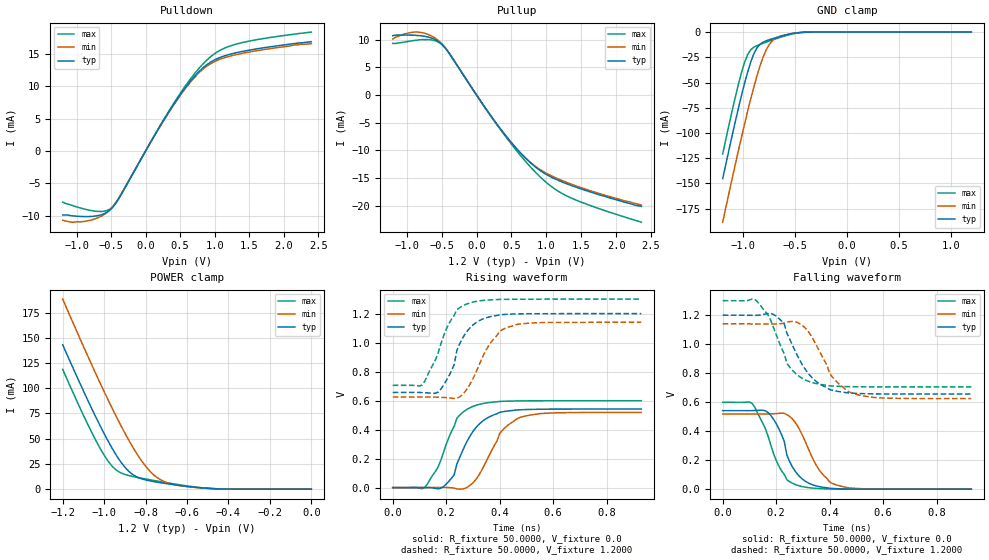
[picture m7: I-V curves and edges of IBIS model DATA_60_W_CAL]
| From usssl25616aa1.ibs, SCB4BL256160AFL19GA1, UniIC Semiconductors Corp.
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|   Model DATA_60_W_CAL
[Model]  DATA_60_W_CAL
Model_type I/O
Polarity   Non-Inverting
Enable   Active-High
Vinl =   0.3800V
Vinh =   0.8200V
Vmeas =  0.6000V
Cref =   5.0000pF
Rref =   50.0000
Vref =   0.6000V
C_comp   1.7430pF   1.7110pF   1.7640pF
[Temperature Range]   25.0000   0.1250k   -40.0000
[Voltage Range]   1.2000V   1.1400V   1.3000V
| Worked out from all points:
|   slope of the pulldown table from 0 to 0.18 V, typ, clamps not added: 54.2 ohm
|   slope of the pullup table from 0 to 0.18 V, typ, clamps not added: 54.6 ohm
|   GND clamp passes 1 mA (typ) near -0.50 V on its own axis
|   POWER clamp passes 1 mA (typ) near -0.51 V on its own axis
|   rising waveform, R_fixture 50.0000, V_fixture 0.0: 20-80 % time 88.7ps typ, 92.8ps min, 78ps max; typ from 0 V to 0.542 V
|   rising waveform, R_fixture 50.0000, V_fixture 1.2000: 20-80 % time 75.5ps typ, 90.2ps min, 83.9ps max; typ from 0.656 V to 1.2 V
|   falling waveform, R_fixture 50.0000, V_fixture 0.0: 20-80 % time 72.3ps typ, 87.4ps min, 80.2ps max; typ from 0.542 V to 0 V
|   falling waveform, R_fixture 50.0000, V_fixture 1.2000: 20-80 % time 98.8ps typ, 96.5ps min, 83.4ps max; typ from 1.2 V to 0.656 V
[Pulldown]
|Voltage   I(typ)   I(min)   I(max)
-1.2V     -9.9mA     -10.7mA    -7.9mA
-1.08V    -10mA      -11mA      -8.35mA
-800mV    -10.12mA   -10.7mA    -9.18mA
-600mV    -9.689mA   -9.814mA   -9.296mA
-480mV    -8.742mA   -8.662mA   -8.678mA
-360mV    -6.833mA   -6.742mA   -6.86mA
400mV     7.094mA    6.992mA    7.231mA
680mV     11.19mA    11.02mA    11.55mA
880mV     13.28mA    13.06mA    13.98mA
1.08V     14.46mA    14.2mA     15.57mA
1.32V     15.21mA    14.92mA    16.54mA
2.4V      16.9mA     16.6mA     18.38mA
[Pullup]
|Voltage   I(typ)   I(min)   I(max)
-1.2V     10.7mA     10.1mA     9.3mA
-1.04V    10.81mA    11mA       9.54mA
-840mV    10.73mA    11.35mA    9.92mA
-680mV    10.41mA    10.85mA    9.979mA
-520mV    9.417mA    9.537mA    9.356mA
-400mV    7.656mA    7.714mA    7.702mA
320mV     -5.719mA   -5.791mA   -5.839mA
600mV     -10.04mA   -10.08mA   -10.46mA
800mV     -12.54mA   -12.46mA   -13.36mA
1.04V     -14.63mA   -14.39mA   -16.21mA
1.28V     -15.97mA   -15.72mA   -18.14mA
2.36V     -20.1mA    -19.9mA    -22.96mA
[GND_clamp]
|Voltage   I(typ)   I(min)   I(max)
-1.2V     -145.3mA   -188.5mA   -120.8mA
-1.05V    -76.2mA    -118.2mA   -52.43mA
-990mV    -51.2mA    -91.62mA   -30.39mA
-960mV    -39.9mA    -78.82mA   -22.48mA
-900mV    -21.67mA   -54.7mA    -15mA
-870mV    -15.78mA   -43.66mA   -13.45mA
-810mV    -10.04mA   -24.79mA   -11.07mA
-780mV    -8.658mA   -17.59mA   -9.958mA
-720mV    -6.57mA    -8.545mA   -7.793mA
-630mV    -3.906mA   -3.64mA    -4.741mA
-420mV    -215.4uA   -240.5uA   -235uA
1.2V      1.597nA    22.84nA    1.463nA
[POWER_clamp]
|Voltage   I(typ)   I(min)   I(max)
-1.2V     143mA      188.4mA    118.7mA
-1.1V     97.38mA    141.5mA    73.24mA
-1.04V    71.38mA    114.3mA    48.22mA
-1V       55.04mA    96.69mA    33.64mA
-960mV    40mA       79.65mA    22.42mA
-900mV    21.75mA    55.6mA     14.58mA
-860mV    14.17mA    41.05mA    12.52mA
-800mV    9.133mA    22.79mA    10.12mA
-740mV    6.786mA    10.88mA    7.886mA
-660mV    4.332mA    4.436mA    5.101mA
-520mV    1.103mA    1.063mA    1.274mA
0V        1.597nA    6.003nA    2.16nA
[Ramp]
| variable   typ   min   max
dV/dt_r  0.3250/88.8406p   0.3110/95.6462p   0.3593/81.8602p
dV/dt_f  0.3264/93.6061p   0.3093/99.0441p   0.3569/86.8204p
R_load = 50.0000
[Rising Waveform]
R_fixture= 50.0000
V_fixture= 0.0
V_fixture_min= 0.0
V_fixture_max= 0.0
|time   V(typ)   V(min)   V(max)
0s        0V         0V         0V
120ps     1.169mV    176.5uV    701uV
170ps     -8.318mV   1.007mV    142.3mV
190ps     6.689mV    1.441mV    243.2mV
230ps     89.65mV    -3.169mV   423.2mV
240ps     162.2mV    -8.685mV   477.9mV
310ps     410.5mV    53.42mV    566.5mV
400ps     518.7mV    373.3mV    594mV
470ps     536mV      479.8mV    597.8mV
930ps     541.6mV    518.3mV    598.9mV
[Rising Waveform]
R_fixture= 50.0000
V_fixture= 1.2000
V_fixture_min= 1.1400
V_fixture_max= 1.3000
|time   V(typ)   V(min)   V(max)
0s        656mV      624.5mV    705.2mV
110ps     655.3mV    624.9mV    706.6mV
170ps     658.9mV    623.3mV    929.9mV
220ps     805mV      616.3mV    1.162V
230ps     848.4mV    614.5mV    1.188V
240ps     946.5mV    617mV      1.226V
280ps     1.082V     685.7mV    1.268V
360ps     1.176V     982mV      1.294V
430ps     1.195V     1.105V     1.298V
930ps     1.2V       1.14V      1.3V
[Falling Waveform]
R_fixture= 50.0000
V_fixture= 0.0
V_fixture_min= 0.0
V_fixture_max= 0.0
|time   V(typ)   V(min)   V(max)
0s        541.6mV    518.3mV    598.9mV
110ps     541.7mV    518mV      591.3mV
170ps     528mV      518.8mV    364mV
220ps     376.8mV    523.7mV    127.6mV
230ps     331.8mV    523.4mV    102.1mV
240ps     234.8mV    513.6mV    65.2mV
280ps     102.4mV    435.8mV    26.5mV
360ps     18.07mV    135.5mV    4.357mV
420ps     3.913mV    32.38mV    895.8uV
930ps     0V         0V         0V
[Falling Waveform]
R_fixture= 50.0000
V_fixture= 1.2000
V_fixture_min= 1.1400
V_fixture_max= 1.3000
|time   V(typ)   V(min)   V(max)
0s        1.2V       1.14V      1.3V
120ps     1.199V     1.139V     1.309V
170ps     1.211V     1.139V     1.2V
200ps     1.193V     1.139V     1.066V
230ps     1.14V      1.145V     934mV
250ps     1.037V     1.155V     842.9mV
330ps     777mV      1.06V      738.1mV
400ps     687mV      798.3mV    712.8mV
480ps     662.5mV    665.4mV    706.7mV
930ps     656mV      624.5mV    705.2mV
